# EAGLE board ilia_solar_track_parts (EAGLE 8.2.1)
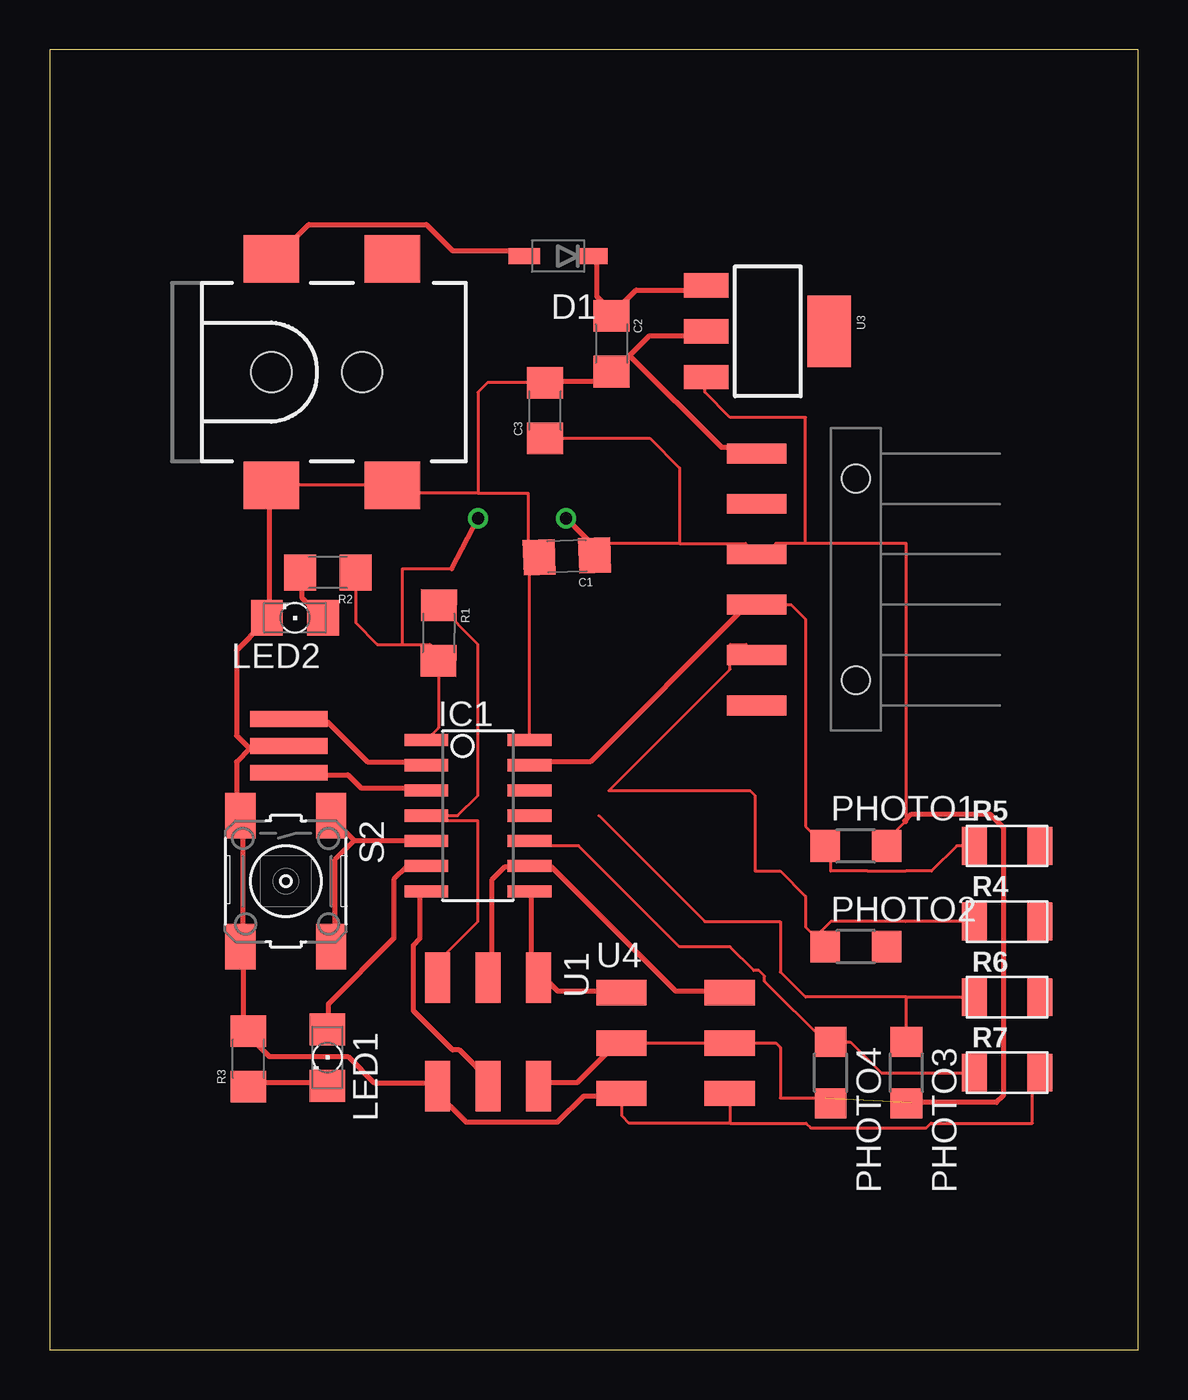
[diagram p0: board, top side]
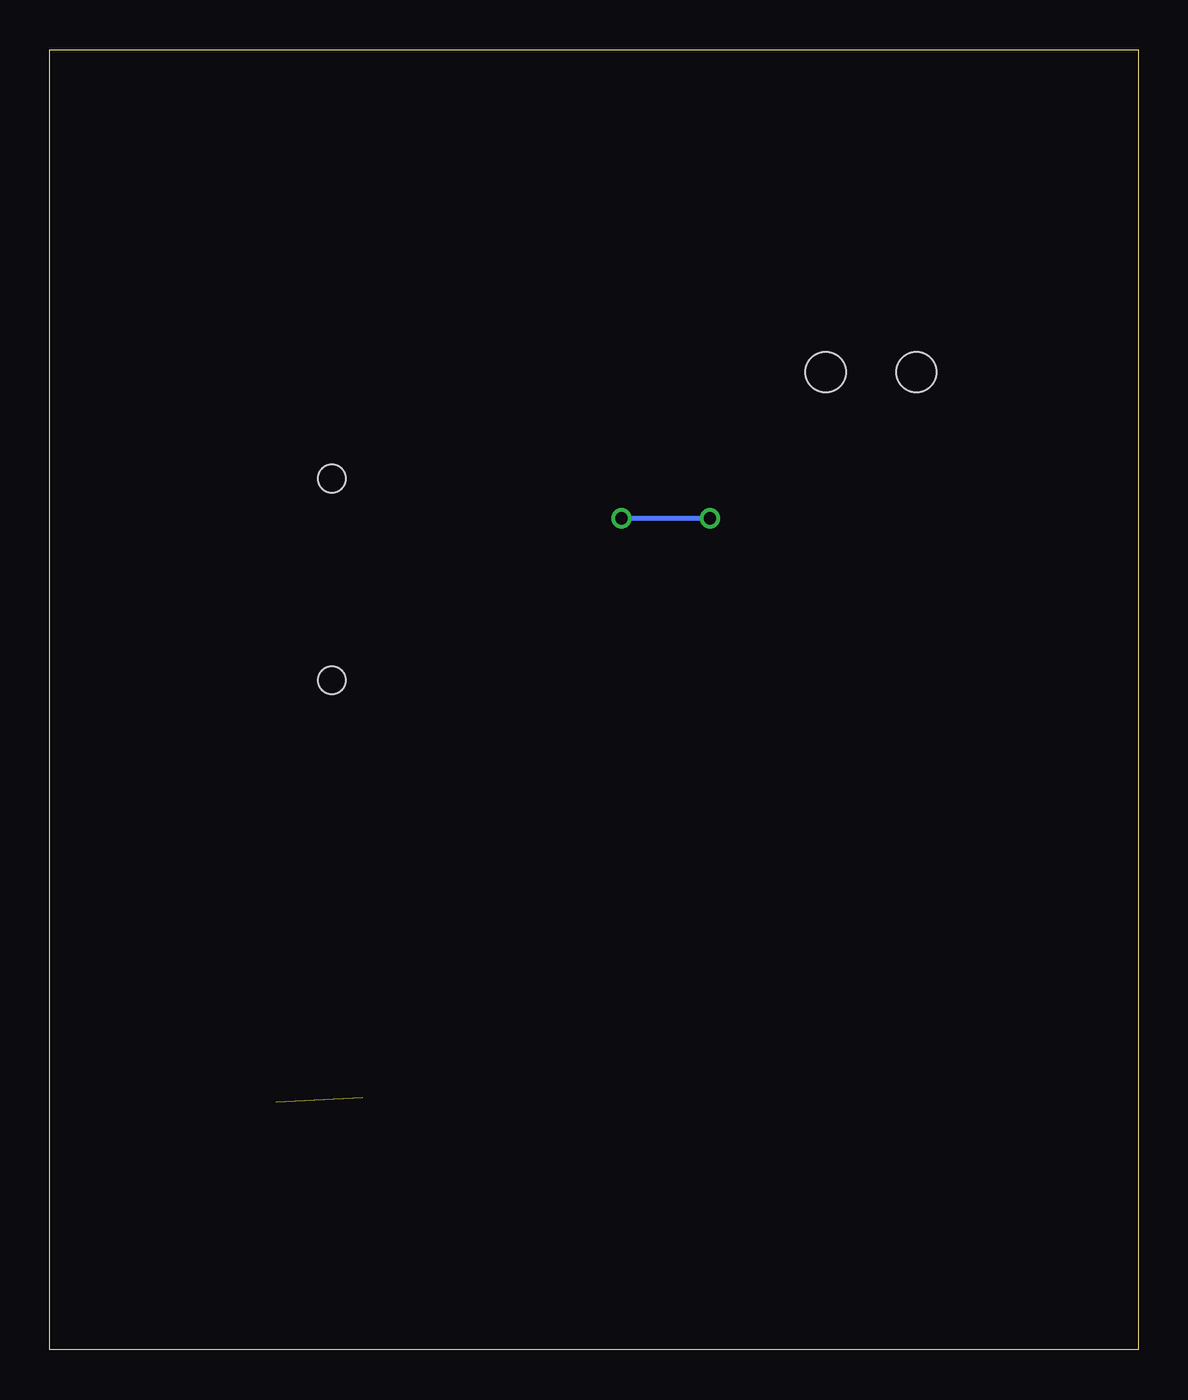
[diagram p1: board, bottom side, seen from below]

Size 54.86 x 65.53 mm. Coordinates in mm from the lower left corner, seen from the top.
Outline: 0,0 54.86,0 54.86,65.53 0,65.52 0,0
Copper layers (1*16): Top 0.035mm / dielectric 1.5mm / Bottom 0.035mm
Design rules "default *": minimum track width 10mil, minimum drill 24mil, track to track 16mil, track to pad 16mil, pad to pad 16mil, via to via 16mil, smd to smd 16mil, copper to edge 40mil, drill to drill 8mil, minimum pad ring 10mil, minimum via ring 8mil, stop-mask expansion 4mil, vias tented up to drill 0mil, thermal gap 10mil

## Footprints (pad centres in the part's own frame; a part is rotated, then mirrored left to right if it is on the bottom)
1206 = smd 1.6 x 1.8: 1 -1.4,0; 2 1.4,0
SOD123 = smd 1.6 x 0.8: ANODE 1.7,0; CATHODE -1.7,0
SOIC14 = smd 0.61 x 2.21: 1 -3.81,-2.603; 2 -2.54,-2.603; 3 -1.27,-2.603; 4 0,-2.603; 5 1.27,-2.603; 6 2.54,-2.603; 7 3.81,-2.603; 8 3.81,2.603; 9 2.54,2.603; 10 1.27,2.603; 11 0,2.603; 12 -1.27,2.603; 13 -2.54,2.603; 14 -3.81,2.603
POWER_JACK_SMD = smd 2.8 x 2.4: GND 0,-5.7; P$4 6.1,-5.7; VIN0 0,5.7; VIN1 6.1,5.7 | hole 2.032: 0,0; 4.572,0
1X06-SMD = smd 1 x 3: 1 -6.35,5; 2 -3.81,5; 3 -1.27,5; 4 1.27,5; 5 3.81,5; 6 6.35,5 | hole 1.4: -5.08,0; 5.08,0
FKIT-LED-1206 = smd 1.6 x 1.803: A -1.422,0; C 1.422,0
OP1206 = smd 1.5 x 1.6: COLLECTOR -1.55,0; EMITTER 1.55,0
R1206FAB = smd 1.27 x 1.905: 1 -1.651,0; 2 1.651,0
6MM_SWITCH = smd 2.286 x 1.524: 1 -3.302,2.286; 2 3.302,2.286; 3 -3.302,-2.286; 4 3.302,-2.286
2X03SMD = smd 2.54 x 1.27: 1 -2.54,2.54; 2 2.92,2.54; 3 -2.54,0; 4 2.92,0; 5 -2.54,-2.54; 6 2.92,-2.54
EFOBM = smd 0.8 x 3.9: 1 -1.35,0; 2 0,0; 3 1.35,0
SOT223 = smd 1.219 x 2.235: 1 -2.311,-3.099; 2 0,-3.099; 3 2.311,-3.099 | smd 3.6 x 2.2: 4 0,3.099

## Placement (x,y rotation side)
C1  0.1uF  [1206]  26.07,39.99 181.8 top
C2  10uF  [1206]  28.31,50.71 270 top
C3  10uF  [1206]  24.97,47.34 90 top
D1  [SOD123]  25.62,55.13 180 top
IC1  ATTINY44-SSU  [SOIC14]  21.59,26.92 270 top
J2  POWER_JACKSMD  [POWER_JACK_SMD]  11.18,49.28 0 top
JP1  [1X06-SMD]  40.64,38.83 90 top
LED1  [FKIT-LED-1206]  14,14.73 270 top
LED2  [FKIT-LED-1206]  12.37,36.9 180 top
PHOTO1  PHOTOTRANSISTOR-NPN1206  [OP1206]  40.64,25.4 0 top
PHOTO2  PHOTOTRANSISTOR-NPN1206  [OP1206]  40.64,20.32 0 top
PHOTO3  PHOTOTRANSISTOR-NPN1206  [OP1206]  43.18,13.97 270 top
PHOTO4  PHOTOTRANSISTOR-NPN1206  [OP1206]  39.37,13.97 270 top
R1  10K  [1206]  19.61,36.13 269.6 top
R2  1K  [1206]  14.02,39.17 180 top
R3  1K  [1206]  10.02,14.67 90 top
R4  10k  [R1206FAB]  48.26,21.59 0 top
R5  10k  [R1206FAB]  48.26,25.4 0 top
R6  10k  [R1206FAB]  48.26,17.78 0 top
R7  10k  [R1206FAB]  48.26,13.97 0 top
S2  [6MM_SWITCH]  11.91,23.62 270 top
U1  AVRISPSMD  [2X03SMD]  22.1,16.22 270 top
U2  RESONATOR  [EFOBM]  12.05,30.44 270 top
U3  V_REG_MIC2920  [SOT223]  36.2,51.34 270 top
U4  AVRISPSMD  [2X03SMD]  31.36,15.46 0 top

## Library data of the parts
C1-C3 J2 JP1 LED1 LED2 R1-R3 U3 = SparkFun
D1 IC1 PHOTO1-PHOTO4 R4-R7 S2 U1 U2 U4 = fab

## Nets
GND: C1.2 C2.2 C3.2 IC1.14 J2.GND J2.P$4 JP1.6 LED2.C R3.2 S2.3 S2.4 U1.6 U2.2 U3.2 U4.5 U4.6
MISO: IC1.8 U1.1 U4.1
MOSI: IC1.7 U1.4
N$1: IC1.2 U2.1
N$2: IC1.3 U2.3
N$3: IC1.6 LED1.A
N$4: D1.ANODE J2.VIN0
N$5: IC1.4 R1.1 U1.5
N$7: PHOTO3.COLLECTOR R6.1
N$8: IC1.5 S2.1 S2.2
N$9: LED1.C R3.1
N$10: C2.1 D1.CATHODE U3.1
N$11: LED2.A R2.2
N$12: PHOTO4.COLLECTOR R7.1
N$13: IC1.11
N$15: IC1.10
N$18: IC1.13
N$19: IC1.12
RX: JP1.2 PHOTO2.COLLECTOR R4.1
SCK: IC1.9 U1.3 U4.2
TX: JP1.3 PHOTO1.COLLECTOR R5.1
VCC: C1.1 C3.1 IC1.1 JP1.4 R1.2 R2.1 U1.2 U3.3 U4.3 U4.4

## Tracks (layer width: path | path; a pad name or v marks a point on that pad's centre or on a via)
GND
  Top 0.152: J2.GND J2.P$4 17.67,43.18 21.59,43.18 | C3.2 22.07,48.74 21.59,48.26 21.59,43.18 | 21.59,43.18 24.13,43.18 24.13,40.64 24.13,40.56 | U4.5 28.82,11.82 29.21,11.43 34.29,11.43 | 49.53,13.59 49.53,11.43 44.42,11.43 44.18,11.19 40.37,11.19 38.37,11.19 38.13,11.43 34.29,11.43 | U4.6 34.28,11.44 34.29,11.43 | IC1.14 24.19,39.49 C1.2
  Top 0.254: 10.08,30.3 9.42,29.64 9.42,27 S2.3 9.75,26.67 9.75,20.4 S2.4 9.75,20.07 9.75,16.1 R3.2 10.08,15.77 11.07,14.78 15.04,14.78 16.36,13.46 19.33,13.46 U1.6 19.33,13.13 20.98,11.48 25.6,11.48 26.92,12.8 28.57,12.8 U4.5 | 10.08,30.3 11.73,30.3 U2.2 | C3.2 25.27,48.79 27.91,48.79 28.24,49.12 C2.2 28.57,49.45 29.23,50.11 | 29.23,50.11 30.23,51.11 32.87,51.11 U3.2 | 29.23,50.11 33.86,45.49 35.51,45.49 JP1.6 | J2.GND 11.07,43.51 11.07,36.91 LED2.C 10.74,36.58 9.42,35.25 9.42,30.96 10.08,30.3 | 24.13,40.64 24.13,40 C1.2
MISO
  Top 0.254: IC1.8 24.28,23.04 24.28,19.41 24.61,19.07 U1.1 24.94,18.75 25.6,18.09 28.57,18.09 U4.1
MOSI
  Top 0.254: IC1.7 18.67,23.04 18.67,20.73 18.34,20.4 18.34,17.09 20.32,15.11 20.65,15.11 22.3,13.46 U1.4
N$1
  Top 0.254: IC1.2 18.67,29.64 16.03,29.64 14.05,31.62 12.07,31.62 U2.1
N$2
  Top 0.254: IC1.3 18.67,28.32 15.7,28.32 15.04,28.98 12.07,28.98 U2.3
N$3
  Top 0.254: LED1.A 14.05,16.43 14.05,17.42 17.35,20.73 17.35,23.7 18.01,24.36 18.67,24.36 IC1.6
N$4
  Top 0.254: D1.ANODE 23.62,55.4 20.32,55.4 19,56.72 13.06,56.72 11.4,55.07 J2.VIN0
N$5
  Top 0.152: U1.5 19.56,19.56 21.59,21.59 21.59,26.67 19.24,26.67 IC1.4 20.57,26.92 21.59,27.94 21.59,35.56 R1.1
N$7
  Top 0.152: 27.69,26.92 33.02,21.59 36.83,21.59 36.83,19.05 38.1,17.78 43.18,17.78 | 43.18,17.78 R6.1 | PHOTO3.COLLECTOR 43.18,17.78
N$8
  Top 0.254: 15.37,25.68 18.67,25.68 IC1.5 | 15.37,25.68 14.38,26.67 S2.1 | 15.37,25.68 14.38,24.69 14.38,20.4 S2.2
N$9
  Top 0.254: R3.1 10.08,13.46 13.72,13.46 LED1.C
N$10
  Top 0.254: D1.CATHODE 27.58,55.07 27.58,53.09 28.24,52.43 C2.1 28.57,52.43 29.57,53.42 32.87,53.42 U3.1
N$11
  Top 0.254: R2.2 12.72,38.89 12.72,37.9 13.72,36.91 LED2.A
N$12
  Top 0.152: PHOTO4.COLLECTOR 40.36,15.52 41.91,13.97 R7.1
N$15
  Top 0.152: IC1.10 24.45,25.4 26.67,25.4 31.75,20.32 34.29,20.32 35.49,19.12 35.75,19.12 36.04,18.84 36.04,18.57 39.09,15.52
RX
  Top 0.152: JP1.2 35.1,35.56 34.29,35.56 34.29,34.29 28.19,28.19 35.31,28.19 35.56,27.94 35.56,24.13 36.83,24.13 38.1,22.86 38.1,21.31 38.59,20.81 | 38.59,20.81 PHOTO2.COLLECTOR | R4.1 43.15,21.59 43.14,21.6 39.38,21.6 38.59,20.81
SCK
  Top 0.254: U1.3 22.3,19.07 22.3,23.7 22.96,24.36 23.95,24.36 IC1.9 24.28,24.36 25.27,24.36 31.55,18.09 34.19,18.09 U4.2
TX
  Top 0.152: R5.1 45.72,25.4 44.45,24.13 43.15,24.13 43.14,24.12 41.24,24.12 41.23,24.13 39.37,24.13 39.37,25.12 PHOTO1.COLLECTOR 38.1,26.39 38.1,36.83 37.37,37.56 JP1.3
  Top 0.254: 24.28,29.64 27.25,29.64 34.85,37.24 35.51,37.24 JP1.3
VCC  (via drill 0.61)  (1 unrouted)
  Top 0.152: 38.1,40.64 36.6,40.64 36.08,40.12 | R2.1 15.42,36.65 16.51,35.56 17.78,35.56 | 17.78,35.56 19.16,35.56 R1.2 19.6,31.35 IC1.1 | 17.78,35.56 17.78,39.37 20.26,39.37 | U4.3 U4.4 36.61,15.46 36.83,15.24 36.83,12.7 39.09,12.7 | 38.1,40.64 38.1,46.99 34.29,46.99 33.02,48.26 33.02,48.94 U3.3 | 42.19,25.68 43.14,26.63 43.18,26.67 43.18,40.64 38.1,40.64 | C3.1 30.26,45.94 31.75,44.45 31.75,40.64 | 31.75,40.64 35.08,40.64 35.84,39.88 | 31.75,40.64 28.1,40.64 C1.1
  Top 0.254: 36.08,40.12 35.84,39.88 JP1.4 | U3.3 33.2,48.79 | U1.2 24.94,13.46 26.59,13.46 28.57,15.44 U4.3 | 43.43,12.47 47.73,12.47 48.06,12.8 48.06,26.34 47.4,27 43.43,27 43.1,26.67 43.14,26.63 | v21.59,41.91 20.26,39.37 | v26.04,41.91 27.3,40.64 C1.1
  Bottom 0.254: v26.04,41.91 v21.59,41.91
